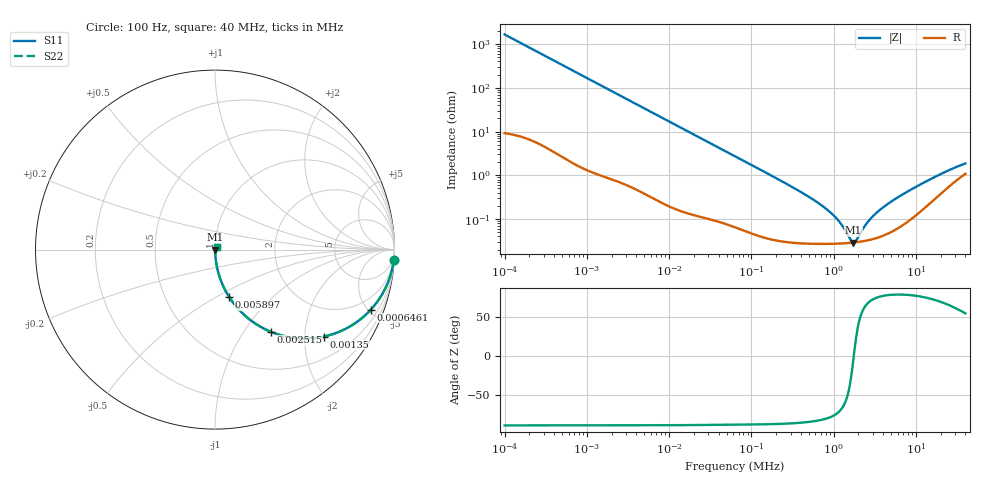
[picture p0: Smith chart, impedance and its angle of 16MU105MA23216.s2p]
!Components F PML CAP
!CONCATENATE F 0.1-40000kHz, at 20deg DC=0V
!Part Number F 16MU105MA23216
!Copyright(C) Rubycon Corporation. 20161128
# MHz S MA R 50
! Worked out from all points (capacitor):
!   561 points, 100 Hz to 40 MHz, reference 50 ohm
!   read as one part in series: C = 961 nF near 104.7 Hz
!   lowest |Z| = 29.1 mohm at 1.744 MHz (marker M1)
!   series resonance near 1.761 MHz, so ESL is about 8.5 nH
!   S11 on the Smith chart (normalised r, x): 100 Hz: 1, -33; 646.1 Hz: 1.04, -5.18; 1.35 kHz: 1.02, -2.48; 2.515 kHz: 1.01, -1.34; 5.897 kHz: 1.01, -0.57; 40 MHz: 1.02, +0.03
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0.0001  0.9978 -3.5  0.0603 86.2  0.0603 86.2  0.9978 -3.5
0.0002692515  0.9859 -9.2  0.1595 80.4  0.1595 80.4  0.9859 -9.2
0.0006460974  0.9304 -21.1  0.3594 68.5  0.3594 68.5  0.9304 -21.1
0.0008716573  0.8842 -27.4  0.4603 62.2  0.4603 62.2  0.8842 -27.4
0.001350255  0.7757 -38.6  0.6246 50.9  0.6246 50.9  0.7757 -38.6
0.002514867  0.5536 -55.8  0.8271 33.6  0.8271 33.6  0.5536 -55.8
0.003806985  0.4038 -65.6  0.9104 23.8  0.9104 23.8  0.4038 -65.6
0.005897271  0.2753 -73.4  0.9583 16.0  0.9583 16.0  0.2753 -73.4
0.007424854  0.2222 -76.5  0.9725 12.8  0.9725 12.8  0.2222 -76.5
0.01865671  0.09086 -84.0  0.9946 5.2  0.9946 5.2  0.09086 -84.0
0.06324555  0.02724 -87.1  0.999 1.6  0.999 1.6  0.02724 -87.1
0.5512845  0.002869 -84.4  0.9997 0.2  0.9997 0.2  0.002869 -84.4
1.0507  0.001104 -75.6  0.9997 0.1  0.9997 0.1  0.001104 -75.6
1.292742  0.0006814 -65.9  0.9997 0.0  0.9997 0.0  0.0006814 -65.9
1.627604  0.0003264 -28.5  0.9997 0.0  0.9997 0.0  0.0003264 -28.5
1.744053  0.0002912 -3.6  0.9997 0.0  0.9997 0.0  0.0002912 -3.6
1.868834  0.0003178 21.9  0.9997 -0.0  0.9997 -0.0  0.0003178 21.9
2.352922  0.0006622 61.6  0.9997 -0.0  0.9997 -0.0  0.0006622 61.6
2.829026  0.001032 70.8  0.9997 -0.1  0.9997 -0.1  0.001032 70.8
4.69589  0.002308 78.0  0.9995 -0.1  0.9995 -0.1  0.002308 78.0
14.51771  0.007877 73.4  0.9978 -0.4  0.9978 -0.4  0.007877 73.4
40  0.01845 53.6  0.9892 -0.9  0.9892 -0.9  0.01845 53.6
